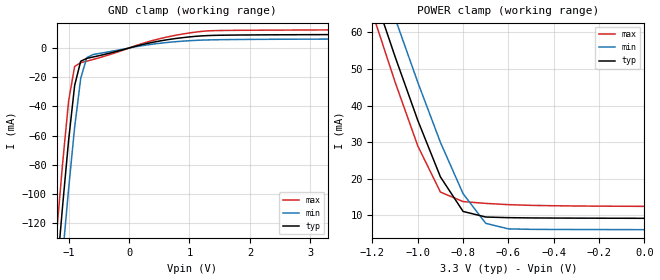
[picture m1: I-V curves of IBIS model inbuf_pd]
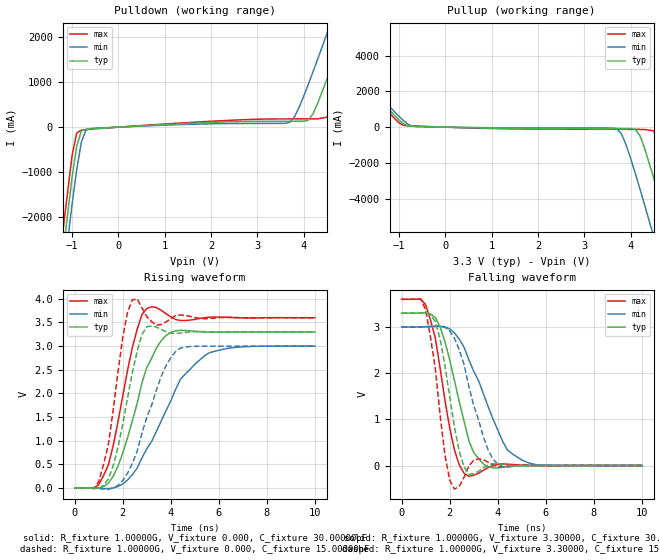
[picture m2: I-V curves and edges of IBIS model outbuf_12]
| IBIS file 2309NZ.ibs created by s2ibis2 version 1.2
| North Carolina State University Electronics Research Laboratory  1995
[IBIS ver]   2.1
[File name]   idt2309nz.ibs
[File Rev]   1.0
[Date]   Wednesday, February 12, 2003 Peter L SDC
[Source]   IDT
[Notes]   1.Temperatures: typ=25C, min=-40C, max=100C
   2.Ramp rates based on 50 ohm load.
[Disclaimer]
READ THESE TERMS AND CONDITIONS CAREFULLY BEFORE USING THIS IBIS MODEL.  BY
USING THIS IBIS MODEL, YOU ARE ACCEPTING AND AGREEING TO THESE TERMS AND
CONDITIONS OF USE.
Integrated Device Technology, Inc. ("IDT") hereby grants the user of this
IBIS model ("User") a non-exclusive, nontransferable license to use this
IBIS model under the following terms: The User is granted this license only
to use the IBIS model for demonstration purposes only and is not granted
rights to sell, copy (except as needed to run the IBIS model), rent, lease
or sub-license (except for demonstration) the IBIS model in whole or in
part, or in modified form to anyone. The User may modify the IBIS model to
suit its specific applications, but  rights to derivative works and such
modifications shall belong to IDT.
THIS IBIS MODEL IS PROVIDED ON AN AS IS" BASIS AND IDT  MAKES ABSOLUTELY NO
WARRANTY WITH RESPECT TO THE INFORMATION CONTAINED HEREIN.  IDT DISCLAIMS
AND USER WAIVES ALL WARRANTIES, EXPRESS AND IMPLIED, INCLUDING WARRANTIES OF
MERCHANTABILITY AND FITNESS FOR A PARTICULAR PURPOSE.  THE ENTIRE RISK AS TO
QUALITY AND PERFORMANCE IS WITH THE USER  ACCORDINGLY, IN NO EVENT SHALL IDT
BE LIABLE FOR ANY DIRECT OR INDIRECT DAMAGES, WHETHER IN CONTRACT OR TORT,
INCLUDING ANY LOST PROFITS OR OTHER INCIDENTAL, CONSEQUENTIAL, EXEMPLARY, OR
PUNITIVE DAMAGES ARISING OUT OF THE USE OR APPLICATION OF THE  IBIS MODEL,
WHETHER OR NOT IDT HAD NOTICE OF SUCH DAMAGES.
IDT reserves the right to make changes without notice to any product herein
to improve reliability, function, or design. IDT does not convey any license
under patent rights or any other intellectual property rights, including those
of third parties. IDT is not obligated to provide maintenance or support for
the licensed IBIS model.
This model is for NINE OUTPUT 3.3V CLOCK BUFFER
[Copyright]
Copyright 2002, Integrated Device Technology, Inc. All rights reserved.
|   Component IDT2309NZ
[Component]   IDT2309NZ
[Manufacturer]   Integrated Device Technology
[Package]
|SO16-10 (Thin Shrink Size Outline Package)
| variable   typ   min   max
R_pkg   52.59000m   52.19000m   52.96000m
L_pkg   4.36000nH   3.91000nH   4.78000nH
C_pkg   0.23700pF   0.15300pF   0.29000pF
|SO16-8 (Small Outline Package)
| variable   typ   min   max
|R_pkg   53.14000m   52.77000m   53.55000m
|L_pkg   5.18000nH   4.04000nH   6.38000nH
|C_pkg   0.38000pF   0.22400pF   0.55100pF
[Pin]  signal_name   model_name   R_pin   L_pin   C_pin
1   BUF_IN   inbuf_pd
2   OUTPUT1   outbuf_12
3   OUTPUT2   outbuf_12
4   VDD   POWER
5   GND   GND
6   OUTPUT3   outbuf_12
7   OUTPUT4   outbuf_12
8   VDD   POWER
9   GND   GND
10   OUTPUT5   outbuf_12
11   OUTPUT6   outbuf_12
12   GND   GND
13   VDD   POWER
14   OUTPUT7   outbuf_12
15   OUTPUT8   outbuf_12
16   OUTPUT9   outbuf_12
| Models and submodels in the file (2): inbuf_pd (Input), outbuf_12 (Output)
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| d   d   dummy_model
|   Model inbuf_pd
[Model]   inbuf_pd
Model_type   Input
Vinl =  0.80000V
Vinh =  2.00000V
C_comp   7.00000pF   7.00000pF   7.00000pF
[Temperature Range]   25.00000   100.00000   -40.00000
[Voltage Range]   3.30000V   3.00000V   3.60000V
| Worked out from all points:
|   GND clamp passes 1 mA (typ) near -0.09 V on its own axis
[GND_clamp]
| voltage   I(typ)   I(min)   I(max)
-3.3V     -1.25A     -1.269A    -1.236A
-1.2V     -156.4mA   -190.2mA   -127.5mA
-1.1V     -108.3mA   -142.3mA   -79.3mA
-1V       -63.1mA    -96.36mA   -36.22mA
-900mV    -25.54mA   -54.09mA   -12.56mA
-800mV    -9.055mA   -20.79mA   -10.08mA
-700mV    -7.093mA   -6.636mA   -9.006mA
-600mV    -6.182mA   -4.511mA   -7.897mA
400mV     3.97mA     2.691mA    5.244mA
1.1V      7.98mA     5.225mA    10.88mA
1.5V      8.732mA    5.694mA    11.97mA
3.3V      9.176mA    6.112mA    12.39mA
[POWER_clamp]
| voltage   I(typ)   I(min)   I(max)
-3.3V     532.9mA    506.2mA    584.5mA
-1.2V     71.61mA    81.89mA    65.25mA
-1.1V     53.31mA    63.82mA    46.38mA
-1V       35.94mA    46.35mA    28.96mA
-900mV    20.48mA    29.92mA    16.33mA
-800mV    11.05mA    15.89mA    13.75mA
-700mV    9.525mA    7.794mA    13.25mA
-600mV    9.351mA    6.286mA    12.91mA
0V        9.176mA    6.074mA    12.44mA
|   Model outbuf_12
[Model]   outbuf_12
Model_type   Output
Polarity   Non-Inverting
Vmeas =  1.65000V
C_comp   7.00000pF   7.00000pF   7.00000pF
[Temperature Range]   25.00000   100.00000   -40.00000
[Voltage Range]   3.30000V   3.00000V   3.60000V
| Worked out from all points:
|   slope of the pulldown table from 0 to 0.495 V, typ, clamps not added: 16.9 ohm
|   slope of the pullup table from 0 to 0.495 V, typ, clamps not added: 16.8 ohm
|   rising waveform, R_fixture 1.00000G, V_fixture 0.000, C_fixture 30.00000pF: 20-80 % time 1.15ns typ, 1.82ns min, 847ps max; typ from 0 V to 3.3 V
|   rising waveform, R_fixture 1.00000G, V_fixture 0.000, C_fixture 15.00000pF: 20-80 % time 788ps typ, 1.18ns min, 611ps max; typ from 0 V to 3.3 V
|   falling waveform, R_fixture 1.00000G, V_fixture 3.30000, C_fixture 30.00000pF: 20-80 % time 918ps typ, 1.42ns min, 698ps max; typ from 3.3 V to 0 V
|   falling waveform, R_fixture 1.00000G, V_fixture 3.30000, C_fixture 15.00000pF: 20-80 % time 629ps typ, 953ps min, 522ps max; typ from 3.3 V to 0 V
[Pulldown]
| voltage   I(typ)   I(min)   I(max)
-3.3V     -22.38A    -22.9A     -21.96A
-1.3V     -3.682A    -4.288A    -3.174A
-1V       -1.118A    -1.712A    -633.7mA
-900mV    -423.4mA   -946.5mA   -130.5mA
-800mV    -83.29mA   -335.1mA   -68.01mA
-700mV    -45.92mA   -66.76mA   -55.61mA
3.7V      129.9mA    105.6mA    182.2mA
4.1V      152mA      949.7mA    183.1mA
4.5V      1.057A     2.067A     218.7mA
4.9V      2.194A     3.221A     1.21A
5.3V      3.358A     4.388A     2.364A
6.6V      7.214A     8.241A     6.219A
[Pullup]
| voltage   I(typ)   I(min)   I(max)
-3.3V     7.061A     7.246A     6.91A
-2.7V     5.286A     5.477A     5.129A
-900mV    183mA      361.9mA    95.61mA
3.7V      -80.26mA   -86.46mA   -121.8mA
3.9V      -82.72mA   -970.8mA   -122.7mA
4.2V      -464.4mA   -3.44A     -127.5mA
4.5V      -2.846A    -6.132A    -202.5mA
4.7V      -4.641A    -7.966A    -1.494A
4.9V      -6.476A    -9.816A    -3.254A
5.1V      -8.331A    -11.67A    -5.087A
5.3V      -10.2A     -13.54A    -6.947A
6.6V      -22.47A    -25.79A    -19.24A
[Ramp]
| variable   typ   min   max
dV/dt_r   1.43520/0.70239n   1.07400/1.14766n   1.73280/0.48226n
dV/dt_f   1.47066/0.43116n   1.23780/0.90175n   1.67964/0.26686n
R_load = 50.00000
[Rising Waveform]
R_fixture = 1.00000G
V_fixture = 0.000
V_fixture_min = 0.000
V_fixture_max = 0.000
C_fixture = 30.00000pF
R_dut = 52.60000m
L_dut = 4.36000nH
C_dut = 0.23700pF
| time   V(typ)   V(min)   V(max)
0s        0V         0V         0V
800ps     -5.921mV   -521uV     -6.464mV
1.4ns     101.6mV    -14.11mV   489.4mV
1.8ns     462.2mV    31.33mV    1.401V
2.4ns     1.425V     281.6mV    2.975V
3ns       2.546V     828.4mV    3.795V
4ns       3.288V     1.844V     3.619V
4.4ns     3.332V     2.297V     3.541V
5.6ns     3.295V     2.857V     3.611V
10ns      3.299V     2.999V     3.599V
[Rising Waveform]
R_fixture = 1.00000G
V_fixture = 0.000
V_fixture_min = 0.000
V_fixture_max = 0.000
C_fixture = 15.00000pF
R_dut = 52.60000m
L_dut = 4.36000nH
C_dut = 0.23700pF
| time   V(typ)   V(min)   V(max)
0s        0V         0V         0V
1ns       -12.61mV   -9.445mV   138.2mV
1.4ns     192.8mV    -25.57mV   920.6mV
1.6ns     467.9mV    -1.196mV   1.644V
2ns       1.355V     159.8mV    3.194V
2.4ns     2.446V     523.3mV    3.979V
3ns       3.407V     1.493V     3.623V
3.8ns     3.303V     2.587V     3.51V
4.4ns     3.277V     2.957V     3.658V
10ns      3.299V     2.999V     3.599V
[Falling Waveform]
R_fixture = 1.00000G
V_fixture = 3.30000
V_fixture_min = 3.00000
V_fixture_max = 3.60000
C_fixture = 30.00000pF
R_dut = 52.60000m
L_dut = 4.36000nH
C_dut = 0.23700pF
| time   V(typ)   V(min)   V(max)
0s        3.299V     2.999V     3.599V
1ns       3.306V     3.002V     3.481V
1.4ns     3.205V     3.012V     2.767V
1.6ns     3.004V     3.014V     2.114V
2.2ns     1.837V     2.87V      335.3mV
2.6ns     960.1mV    2.56V      -168.3mV
3ns       281.2mV    2.043V     -209.8mV
3.4ns     34.76mV    1.562V     -104.2mV
4.6ns     -11.33mV   255.7mV    23.24mV
10ns      55.77uV    180.2uV    23.99uV
[Falling Waveform]
R_fixture = 1.00000G
V_fixture = 3.30000
V_fixture_min = 3.00000
V_fixture_max = 3.60000
C_fixture = 15.00000pF
R_dut = 52.60000m
L_dut = 4.36000nH
C_dut = 0.23700pF
| time   V(typ)   V(min)   V(max)
0s        3.299V     2.999V     3.599V
1ns       3.312V     3.005V     3.371V
1.4ns     3.119V     3.022V     2.108V
1.6ns     2.744V     3.021V     1.1V
2ns       1.493V     2.914V     -312.2mV
2.2ns     832mV      2.752V     -511.9mV
2.8ns     -184.8mV   1.711V     -8.356mV
3.6ns     9.38mV     339.9mV    72.92mV
4ns       42.31mV    32.38mV    -24.12mV
10ns      45.11uV    127.6uV    -11.65uV
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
